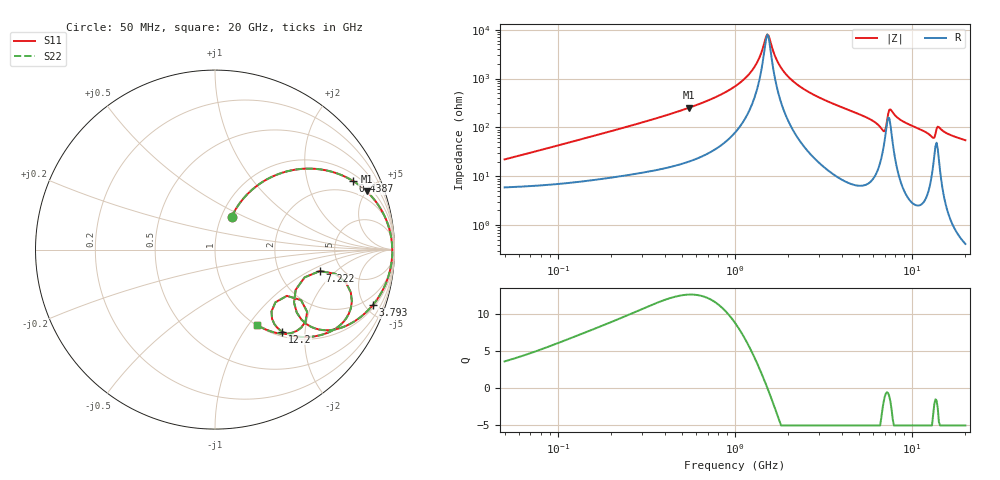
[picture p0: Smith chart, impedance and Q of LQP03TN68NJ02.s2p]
!Murata Part Number: LQP03TN68NJ02
!These Parameters are Measured in Series Mode Connection
!  o--[Z]--o
!Port1  Port2
!  o-------o
!Freq. Start=50[MHz] Stop=20[GHz], 401[Steps]
# Hz S RI R 50
!Freq.(Hz) S11(Real) S11(Imag) S21(Real) S21(Imag) S12(Real) S12(Imag) S22(Real) S22(Imag)
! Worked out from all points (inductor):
!   401 points, 50 MHz to 20 GHz, reference 50 ohm
!   read as one part in series: L = 67.5 nH near 51.52 MHz
!   highest Q = 12.6 at 549.3 MHz (marker M1), where L = 72.9 nH
!   self-resonance near 1.521 GHz
!   S11 on the Smith chart (normalised r, x): 50 MHz: 1.12, +0.43; 438.7 MHz: 1.31, +3.83; 3.793 GHz: 1.19, -5.61; 7.222 GHz: 3.44, -1.28; 12.2 GHz: 1.08, -1.53; 20 GHz: 1.01, -1.09
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5e7  0.0927 0.1829  0.9073 -0.1829  0.9073 -0.1829  0.0927 0.1829
1.364002e8  0.2761 0.3839  0.7239 -0.3839  0.7239 -0.3839  0.2761 0.3839
3.721004e8  0.7026 0.416  0.2974 -0.416  0.2974 -0.416  0.7026 0.416
4.387496e8  0.7689 0.3825  0.2311 -0.3825  0.2311 -0.3825  0.7689 0.3825
5.492803e8  0.8454 0.3239  0.1546 -0.3239  0.1546 -0.3239  0.8454 0.3239
1e9  0.9647 0.1362  0.0353 -0.1362  0.0353 -0.1362  0.9647 0.1362
1.270815e9  0.9829 0.0589  0.0171 -0.0589  0.0171 -0.0589  0.9829 0.0589
1.521052e9  0.9877 0.000994  0.0123 -0.000994  0.0123 -0.000994  0.9877 0.000994
1.740566e9  0.9865 -0.0427  0.0135 0.0427  0.0135 0.0427  0.9865 -0.0427
1.904239e9  0.9833 -0.0722  0.0167 0.0722  0.0167 0.0722  0.9833 -0.0722
2.728004e9  0.9497 -0.1935  0.0503 0.1935  0.0503 0.1935  0.9497 -0.1935
3.792786e9  0.8791 -0.3093  0.1209 0.3093  0.1209 0.3093  0.8791 -0.3093
6.217679e9  0.6025 -0.4485  0.3975 0.4485  0.3975 0.4485  0.6025 -0.4485
6.905011e9  0.4402 -0.2949  0.5598 0.2949  0.5598 0.2949  0.4402 -0.2949
7.222371e9  0.5839 -0.1197  0.4161 0.1197  0.4161 0.1197  0.5839 -0.1197
7.442007e9  0.7291 -0.1829  0.2709 0.1829  0.2709 0.1829  0.7291 -0.1829
8.644534e9  0.6577 -0.4487  0.3423 0.4487  0.3423 0.4487  0.6577 -0.4487
1.220001e10  0.3754 -0.4575  0.6246 0.4575  0.6246 0.4575  0.3754 -0.4575
1.354865e10  0.4005 -0.2577  0.5995 0.2577  0.5995 0.2577  0.4005 -0.2577
1.417136e10  0.5042 -0.4018  0.4958 0.4018  0.4958 0.4018  0.5042 -0.4018
1.527346e10  0.3958 -0.469  0.6042 0.469  0.6042 0.469  0.3958 -0.469
2e10  0.2315 -0.418  0.7685 0.418  0.7685 0.418  0.2315 -0.418
